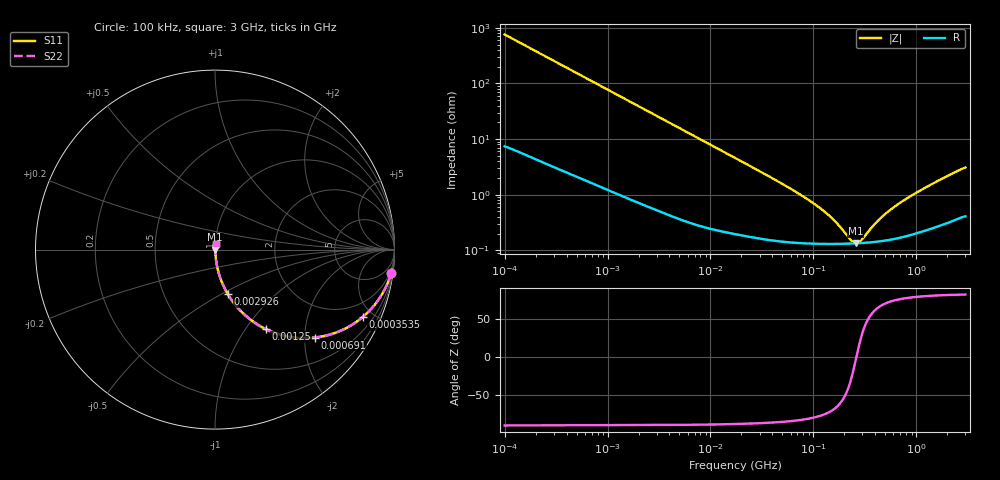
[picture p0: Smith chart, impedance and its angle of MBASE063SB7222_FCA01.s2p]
! MBASE063SB7222_FCA01  S-PARAMETER MODEL  ( Standard Model )
! Model Generated by TAIYO YUDEN Corporation (http://www.ty-top.com)
! Version 1.0
! TAIYO YUDEN Control No. 220601
! Copyright(c) 2020 TAIYO YUDEN CO.,LTD. All Rights Reserved.
! Product Description (link to TY-COMPAS)
! https://ds.yuden.co.jp/TYCOMPAS/or/detail?pn=MBASE063SB7222KFCA01&u=M
! Products Name : Multilayer Ceramic Capacitors
! Characteristics :
!  Capacitance : 2200 [pF] , Rated Voltage : 16 [V] , TCC : X7R
!  Case Size : 0.6 x 0.3 / 0.024 x 0.012 [mm/inch] , Thickness : 0.3 / 0.012 [mm/inch]
!  (Conditions: Temperature = 25 [degC] , DC Bias Voltage = 0 [V])
! External Node Assignments :
!  1  o---| |---o  2
! GND o---------o GND
! Frequency Range : 100kHz  -  3GHz  [ 401 STEP ]
# MHZ S RI R 50
! Freq[MHz].  S11 Real  S11 Imag  S21 Real  S21 Imag  S12 Real  S12 Imag  S22 Real  S22 Imag
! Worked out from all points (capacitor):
!   401 points, 100 kHz to 3 GHz, reference 50 ohm
!   read as one part in series: C = 2.09 nF near 105.3 kHz
!   lowest |Z| = 133 mohm at 259.3 MHz (marker M1)
!   series resonance near 261.5 MHz, so ESL is about 180 pH
!   S11 on the Smith chart (normalised r, x): 100 kHz: 1, -15; 353.5 kHz: 1.06, -4.34; 691 kHz: 1.03, -2.23; 1.25 MHz: 1.02, -1.24; 2.926 MHz: 1.01, -0.54; 3 GHz: 1.01, +0.06
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0.1  0.9818 -0.1289  0.0182 0.1289  0.0182 0.1289  0.9818 -0.1289
0.205778  0.93 -0.2494  0.07 0.2494  0.07 0.2494  0.93 -0.2494
0.353547  0.822 -0.3762  0.178 0.3762  0.178 0.3762  0.822 -0.3762
0.562235  0.6507 -0.4698  0.3493 0.4698  0.3493 0.4698  0.6507 -0.4698
0.690972  0.5545 -0.4898  0.4455 0.4898  0.4455 0.4898  0.5545 -0.4898
0.917447  0.4172 -0.4854  0.5828 0.4854  0.5828 0.4854  0.4172 -0.4854
1.249956  0.2817 -0.4417  0.7183 0.4417  0.7183 0.4417  0.2817 -0.4417
1.887902  0.1501 -0.3483  0.8499 0.3483  0.8499 0.3483  0.1501 -0.3483
2.925885  0.0711 -0.2473  0.9289 0.2473  0.9289 0.2473  0.0711 -0.2473
3.161081  0.0621 -0.2313  0.9379 0.2313  0.9379 0.2313  0.0621 -0.2313
6.848882  0.0159 -0.1131  0.9841 0.1131  0.9841 0.1131  0.0159 -0.1131
17.7727  0.00391 -0.0444  0.9961 0.0444  0.9961 0.0444  0.00391 -0.0444
52.46276  0.00163 -0.0147  0.9984 0.0147  0.9984 0.0147  0.00163 -0.0147
97.38194  0.00136 -0.00713  0.9986 0.00713  0.9986 0.00713  0.00136 -0.00713
147.0833  0.00131 -0.00375  0.9987 0.00375  0.9987 0.00375  0.00131 -0.00375
233.9019  0.00132 -0.000687  0.9987 0.000687  0.9987 0.000687  0.00132 -0.000687
259.3015  0.00133 -5.06e-05  0.9987 5.06e-05  0.9987 5.06e-05  0.00133 -5.06e-05
287.4592  0.00134 0.000584  0.9987 -0.000584  0.9987 -0.000584  0.00134 0.000584
412.3589  0.00143 0.00289  0.9986 -0.00289  0.9986 -0.00289  0.00143 0.00289
547.5153  0.00156 0.00492  0.9984 -0.00492  0.9984 -0.00492  0.00156 0.00492
1097.999  0.00225 0.0117  0.9978 -0.0117  0.9978 -0.0117  0.00225 0.0117
3000  0.00498 0.0303  0.995 -0.0303  0.995 -0.0303  0.00498 0.0303
